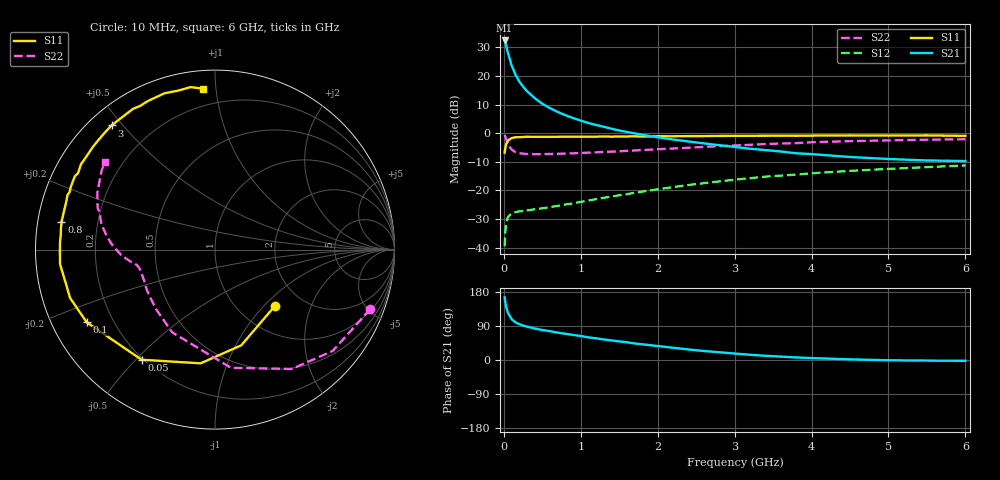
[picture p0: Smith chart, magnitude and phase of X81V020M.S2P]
! SIEMENS Small Signal Semiconductors
! BFP136W
! Si NPN RF Bipolar Junction Transistor in SOT343
! VCE = 1 V  IC = 20 mA
! Common Emitter S-Parameters:  September  1994
# GHz  S  MA  R  50
!  f  S11  S21  S12  S22
! GHz  MAG  ANG  MAG  ANG  MAG  ANG  MAG  ANG
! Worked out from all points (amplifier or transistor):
!   40 points, 10 MHz to 6 GHz, reference 50 ohm
!   highest |S21| = 32.4 dB at 10 MHz (marker M1)
!   |S21| within 3 dB of that: start of sweep to 40.93 MHz
!   unconditionally stable (mu >= 1): 806.8 MHz to 2.955 GHz; 5.816 GHz to end of sweep
!   at 200 MHz: K = 0.35, MSG = 22.7 dB, |S12| = -27.3 dB
!   at 1.5 GHz: K = 1.18, MAG = 8.8 dB, |S12| = -21.7 dB
!   at 6 GHz: K = 1.02, MAG = -0.2 dB, |S12| = -11.3 dB
!   S11 on the Smith chart (normalised r, x): 10 MHz: 1.45, -1.16; 50 MHz: 0.19, -0.52; 100 MHz: 0.10, -0.26; 800 MHz: 0.07, +0.09; 3 GHz: 0.06, +0.47; 6 GHz: 0.10, +0.92
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0.01  0.4581 -43.4  41.83 165.2  0.0106 72.9  0.9266 -21.0
0.02  0.5528 -74.6  37.97 151.7  0.0194 63.5  0.8654 -40.7
0.03  0.6387 -97.2  34.17 141.0  0.0261 53.1  0.791 -57.2
0.05  0.7375 -123.7  26.3 125.7  0.0337 39.5  0.6646 -82.3
0.1  0.8217 -150.5  15.45 107.9  0.0399 26.1  0.519 -117.4
0.15  0.8513 -161.6  10.66 99.6  0.0416 22.8  0.467 -134.6
0.2  0.8526 -167.6  8.061 94.6  0.0431 21.8  0.4478 -144.6
0.25  0.8597 -171.8  6.514 90.8  0.0437 22.2  0.4392 -150.8
0.3  0.8672 -174.7  5.456 88.1  0.0445 23.1  0.4325 -155.0
0.4  0.8641 -179.4  4.11 83.2  0.0469 25.8  0.4298 -160.3
0.5  0.8646 177.2  3.277 79.1  0.0486 28.3  0.4304 -163.7
0.6  0.8632 174.8  2.736 75.9  0.051 31.2  0.4331 -165.6
0.7  0.8664 172.1  2.355 72.2  0.0537 34.4  0.4362 -166.9
0.8  0.8688 169.9  2.063 69.2  0.0568 36.9  0.4406 -168.0
1.1  0.8691 163.5  1.507 59.7  0.0666 42.5  0.4571 -170.3
1.5  0.876 156.6  1.116 49.1  0.0823 47.4  0.4835 -172.8
2.2  0.8844 143.9  0.777 32.2  0.1143 49.4  0.54 -178.8
3  0.9006 129.8  0.575 17.0  0.1541 45.7  0.6105 172.5
3.2  0.9003 126.4  0.536 13.8  0.1636 44.2  0.6272 170.1
4.5  0.9153 107.9  0.384 1.7  0.2196 33.1  0.7273 154.4
5.5  0.9156 98.5  0.334 -1.6  0.2555 25.0  0.7701 145.1
6  0.8983 94.2  0.326 -2.2  0.273 20.5  0.7847 141.3
